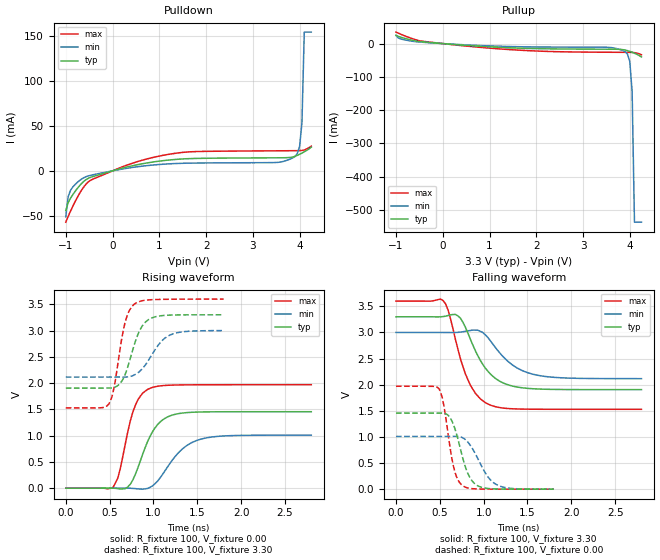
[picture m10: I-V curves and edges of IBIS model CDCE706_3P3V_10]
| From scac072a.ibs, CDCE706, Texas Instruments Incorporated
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|   Model   CDCE706_3P3V_10
[Model]   CDCE706_3P3V_10
Model_type   Output
Polarity   Non-Inverting
Vmeas  =   1.50V
Cref   =   3.00pF
Rref   =   100
Vref   =   0.00V
|Variable   typ   min   max
C_comp   1.493e-12   1.485e-12   1.514e-12
|Variable   typ   min   max
[Voltage range]   3.3   3.0   3.6
|Variable   typ   min   max
[Temperature range]  55   110   -15
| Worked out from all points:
|   slope of the pulldown table from 0 to 0.495 V, typ, clamps not added: 76.7 ohm
|   slope of the pullup table from 0 to 0.495 V, typ, clamps not added: 93.5 ohm
|   rising waveform, R_fixture 100, V_fixture 0.00: 20-80 % time 226ps typ, 299ps min, 169ps max; typ from 0 V to 1.46 V
|   falling waveform, R_fixture 100, V_fixture 3.30: 20-80 % time 277ps typ, 329ps min, 233ps max; typ from 3.3 V to 1.91 V
|   rising waveform, R_fixture 100, V_fixture 3.30: 20-80 % time 168ps typ, 225ps min, 129ps max; typ from 1.91 V to 3.3 V
|   falling waveform, R_fixture 100, V_fixture 0.00: 20-80 % time 152ps typ, 205ps min, 114ps max; typ from 1.46 V to 0.001 V
[Pulldown]
|Voltage   I(typ)   I(min)   I(max)
-1V       -44.26mA   -51.25mA   -57.3mA
-950mV    -35.5mA    -29.01mA   -50.93mA
-900mV    -30.63mA   -21.78mA   -45.1mA
-700mV    -16.26mA   -10.57mA   -24.71mA
-450mV    -6.857mA   -4.753mA   -9.982mA
500mV     6.506mA    4.343mA    9.764mA
1.6V      13.55mA    8.546mA    21.04mA
3.9V      16.23mA    15.94mA    22.49mA
4V        18.48mA    27.22mA    22.61mA
4.05V     19.8mA     53.39mA    22.79mA
4.1V      21.22mA    154.8mA    23.2mA
4.25V     26.49mA    154.8mA    27.61mA
[Pullup]
|Voltage   I(typ)   I(min)   I(max)
-1V       25.06mA    24.17mA    34.52mA
-900mV    19.22mA    13.99mA    28.29mA
-500mV    6.193mA    4.688mA    8.496mA
750mV     -7.645mA   -5.56mA    -10.69mA
2.05V     -15.26mA   -10.17mA   -22.56mA
3.5V      -16.87mA   -11.05mA   -25.99mA
3.9V      -19.37mA   -24.21mA   -26.26mA
3.95V     -21.16mA   -31.29mA   -26.29mA
4V        -23.41mA   -53.83mA   -26.37mA
4.05V     -26.04mA   -144.1mA   -26.59mA
4.1V      -28.98mA   -536.4mA   -27.22mA
4.25V     -40.22mA   -536.4mA   -33.61mA
[Ramp]
|Variable   typ   min   max
dV/dt_r  0.4837/1.829e-10   0.3144/2.458e-10   0.7242/1.414e-10
dV/dt_f  0.4289/2.114e-10   0.2693/2.573e-10   0.6606/1.719e-10
R_load  =  50
[Rising Waveform]
R_fixture   =   100
V_fixture   =   0.00
V_fixture_min   =   0.00
V_fixture_max   =   0.00
C_fixture   =   0.00
|Time   V(typ)   V(min)   V(max)
0s        0V         0V         0V
537.4ps   1.009mV    325.3uV    11.72mV
593.9ps   -7.99mV    1.463mV    196.7mV
707.1ps   25.12mV    1.77mV     1.074V
791.9ps   258.9mV    -7.338mV   1.571V
961.6ps   989.8mV    18.4mV     1.901V
1.16ns    1.356V     403.3mV    1.958V
1.329ns   1.43V      746.8mV    1.966V
1.499ns   1.449V     911.8mV    1.968V
2.8ns     1.456V     1.009V     1.969V
[Falling Waveform]
R_fixture   =   100
V_fixture   =   3.30
V_fixture_min   =   3.00
V_fixture_max   =   3.60
C_fixture   =   0.00
|Time   V(typ)   V(min)   V(max)
0s        3.3V       3V         3.6V
537.4ps   3.304V     3V         3.611V
593.9ps   3.324V     2.999V     3.429V
707.1ps   3.316V     3.002V     2.675V
820.2ps   2.989V     3.03V      2.095V
933.3ps   2.556V     3.043V     1.783V
1.075ns   2.207V     2.845V     1.61V
1.301ns   1.986V     2.414V     1.541V
1.556ns   1.923V     2.203V     1.531V
2.8ns     1.906V     2.116V     1.529V
[Rising Waveform]
R_fixture   =   100
V_fixture   =   3.30
V_fixture_min   =   3.00
V_fixture_max   =   3.60
C_fixture   =   0.00
|Time   V(typ)   V(min)   V(max)
0s        1.905V     2.115V     1.528V
490.9ps   1.906V     2.115V     1.604V
545.5ps   1.915V     2.116V     1.877V
672.7ps   2.148V     2.114V     3.132V
709.1ps   2.321V     2.118V     3.326V
781.8ps   2.733V     2.156V     3.503V
909.1ps   3.162V     2.348V     3.577V
1.055ns   3.274V     2.723V     3.591V
1.164ns   3.292V     2.893V     3.594V
1.8ns     3.299V     2.999V     3.599V
[Falling Waveform]
R_fixture   =   100
V_fixture   =   0.00
V_fixture_min   =   0.00
V_fixture_max   =   0.00
C_fixture   =   0.00
|Time   V(typ)   V(min)   V(max)
0s        1.457V     1.01V      1.97V
490.9ps   1.456V     1.01V      1.923V
545.5ps   1.453V     1.009V     1.605V
654.5ps   1.241V     1.012V     447.2mV
709.1ps   942.7mV    1.01V      170.5mV
763.6ps   582.9mV    981.7mV    62.95mV
890.9ps   115.6mV    722.4mV    7.705mV
1.036ns   16.21mV    264.8mV    1.657mV
1.145ns   4.581mV    88.61mV    944.2uV
1.8ns     595.5uV    744.3uV    637.2uV
